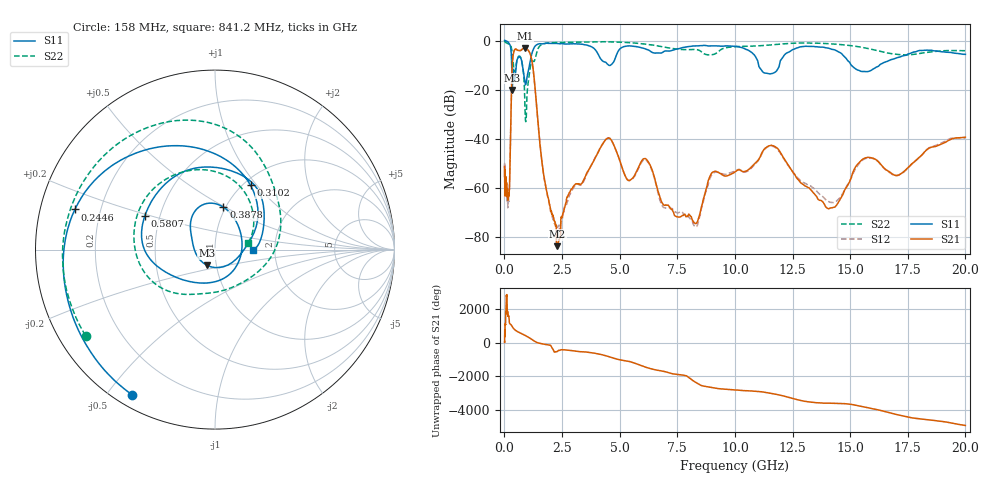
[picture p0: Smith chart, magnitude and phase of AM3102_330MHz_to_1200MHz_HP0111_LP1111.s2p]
! Date/Time: Tue, Sep 11, 2018 5:16 PM
! Network Analyzer: Agilent Technologies E8362B Rev: A.07.50.63
! Sweep from 0.010 to 20.000 GHz, 1601 Points, Sweep Type: LOG
! Power Supply: 4.949 V, 0.001 A
# Hz S DB R 50
!freq MagS11 AngS11 MagS21 AngS21 MagS12 AngS12 MagS22 AngS22
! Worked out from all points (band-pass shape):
!   1601 points, 10 MHz to 20 GHz, reference 50 ohm
!   highest |S21| = -3.05 dB at 890.6 MHz (marker M1); lowest = -83.9 dB at 2.303 GHz (marker M2)
!   |S21| within 3 dB of the highest: 378 MHz to 1.139 GHz (760.9 MHz wide, 100 % of centre)
!   lowest |S11| = -20.2 dB at 341.1 MHz (marker M3), VSWR 1.22, Z = 45 - j7.9 ohm
!   |S11| at or under -10 dB: 779.3 MHz to 1.089 GHz (309.7 MHz wide, 33.2 % of centre); 11.03 GHz to 11.93 GHz (901.6 MHz wide, 7.85 % of centre); 15.04 GHz to 16.28 GHz (1.236 GHz wide, 7.89 % of centre)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
!   |S22| runs from -33.1 to -0.3 dB; largest |S21 - S12| = 0.012
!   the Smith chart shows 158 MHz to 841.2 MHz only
!   S11 on the Smith chart (normalised r, x): 158 MHz: 0.05, -0.58; 244.6 MHz: 0.11, +0.14; 310.2 MHz: 1.08, +0.93; 387.8 MHz: 0.98, +0.49; 580.7 MHz: 0.41, +0.19; 841.2 MHz: 1.53, -0.01
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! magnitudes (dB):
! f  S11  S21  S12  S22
! 10 MHz  0.0  -51.5  -50.2  -0.3
! 35.55 MHz  0.0  -57.1  -60.9  -0.6
! 126.4 MHz  -0.4  -63.3  -64.5  -1.1
! 158 MHz  -0.6  -63.7  -65.2  -1.3
! 244.6 MHz  -1.8  -50.2  -50.3  -1.7
! 310.2 MHz  -7.8  -19.0  -19.0  -3.2
! 341.1 MHz  -20.2  -9.9  -9.9  -5.7
! 387.8 MHz  -12.3  -5.5  -5.6  -9.6
! 447.2 MHz  -16.1  -3.7  -3.8  -12.7
! 580.7 MHz  -7.3  -4.0  -4.1  -7.0
! 841.2 MHz  -13.5  -3.1  -3.2  -14.6
! 890.6 MHz  -17.1  -3.1  -3.1  -27.2
! 1.219 GHz  -4.5  -9.7  -9.7  -8.3
! 1.59 GHz  -1.3  -46.2  -46.1  -1.8
! 2.303 GHz  -1.2  -83.9  -76.2  -0.8
! 4.436 GHz  -9.3  -40.1  -40.0  -0.5
! 5.652 GHz  -2.4  -54.9  -55.3  -1.0
! 6.186 GHz  -3.7  -48.7  -49.2  -1.6
! 8.188 GHz  -2.2  -73.7  -74.8  -3.6
! 11.47 GHz  -13.6  -43.0  -43.2  -1.9
! 14.07 GHz  -3.1  -68.6  -65.7  -1.3
! 20 GHz  -5.6  -39.4  -39.8  -4.2
